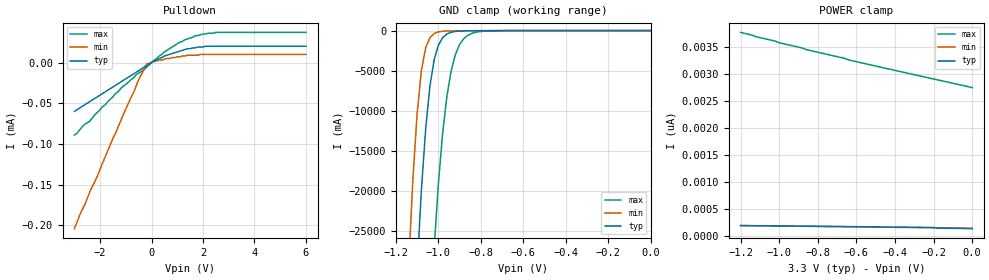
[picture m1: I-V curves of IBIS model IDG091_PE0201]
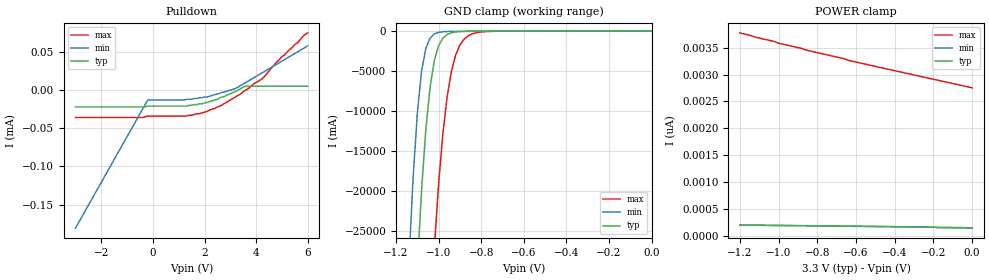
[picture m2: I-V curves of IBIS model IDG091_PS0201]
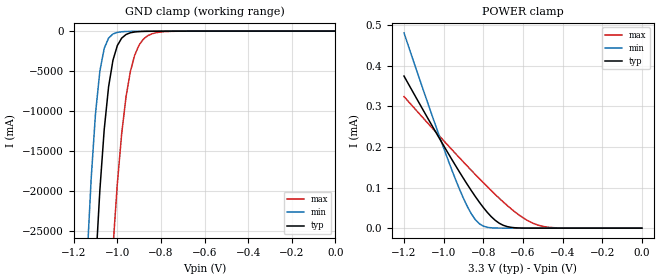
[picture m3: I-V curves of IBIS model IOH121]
| Texas Instruments Incorporated
| DAC5652A DUAL, 10-BIT 275 MSPS DIGITAL-TO-ANALOG CONVERTER
[IBIS Ver]   2.1
[File name]   dac5652a.ibs
[File Rev]   1.0
[Date]   22 FEB 2018
[Source]   Preliminary Model
[Notes]
   Technology type GS30
[Disclaimer]   Please be aware that in the absence of a written agreement
|   Texas Instruments(TI) assumes no liability for:
|   (1) The accuracy of the IBIS models provided to your company
|   (2) The proper functioning of these Models in your design
|   or for any resulting applications;or
|   property rights resulting from your use of these models.
|   TI provides IBIS Models as a service to our customers and
|   therefore reserves the right to limit distribution of the
|   Models.
[Copyright]   Property of Texas Instruments Incorporated.
|   Unauthorised reproduction and/or distribution is strictly.
|   prohibited.
|   This product is protected under copyright law and trade
|   secret law as an unpublished work.
|   (C) Copyright 2018,
|   Texas Instruments Incorporated. All Rights Reserved.
|   These commodities are under the U.S.
|   Government distribution license control.As such,they are not
|   to be re-exported without the prior approval of the U.S.
|   Department of Commerce.
|  Component DAC5652A 48-pin TQFP - PFB Package
|  Part # DAC5652A
[Component]   DAC5652A
[Manufacturer]   Texas Instruments
[Package]   |48 TQFP - PFB Package
|   typ   min   max
R_pkg   0.114   0.028   0.162
L_pkg   3.172nH   2.482nH   4.042nH
C_pkg   0.140pF   0.089pF   0.217pF
[Pin]   signal_name   model_name   R_pin   L_pin   C_pin
   1   DA9   IDG091_PE0201   0.083   3.524nH   0.213pF
   2   DA8   IDG091_PE0201   0.153   3.828nH   0.113pF
   3   DA7   IDG091_PE0201   0.147   3.682nH   0.108pF
   4   DA6   IDG091_PE0201   0.143   3.569nH   0.104pF
   5   DA5   IDG091_PE0201   0.140   3.487nH   0.103pF
   6   DA4   IDG091_PE0201   0.073   3.022nH   0.199pF
   7   DA3   IDG091_PE0201   0.139   3.401nH   0.104pF
   8   DA2   IDG091_PE0201   0.140   2.975nH   0.197pF
   9   DA1   IDG091_PE0201   0.140   3.391nH   0.098pF
   10   DA0   IDG091_PE0201   0.140   3.410nH   0.103pF
   11   NC   nc   0.141   3.461nH   0.105pF
   12   NC   nc   0.073   3.102nH   0.206pF
   13   NC   nc   0.073   3.174nH   0.211pF
   14   NC   nc   0.073   3.260nH   0.218pF
   15   DGND   GND   0.078   3.360nH   0.223pF
   16   DVDD   POWER   0.028   2.456nH   0.090pF
   17   WRTA/WRTIQ   IDG091_PE0201   0.153   3.934nH   0.103pF
   18   CLKA/CLKIQ   IDG091_PE0201   0.076   3.327nH   0.217pF
   19   CLKB/RESETIQ  IDG091_PE0201   0.076   3.233nH   0.212pF
   20   WRTB/SELECTIQ IDG091_PE0201   0.073   3.154nH   0.206pF
   21   DGND   GND   0.073   3.096nH   0.204pF
   22   DVDD   POWER   0.073   3.051nH   0.202pF
   23   DB9   IDG091_PE0201   0.073   3.018nH   0.201pF
   24   DB8   IDG091_PE0201   0.143   3.416nH   0.105pF
   25   DB7   IDG091_PE0201   0.073   2.993nH   0.198pF
   26   DB6   IDG091_PE0201   0.073   3.008nH   0.199pF
   27   DB5   IDG091_PE0201   0.141   3.462nH   0.105pF
   28   DB4   IDG091_PE0201   0.143   3.533nH   0.107pF
   29   DB3   IDG091_PE0201   0.075   3.190nH   0.210pF
   30   DB2   IDG091_PE0201   0.075   3.272nH   0.215pF
   31   DB1   IDG091_PE0201   0.153   3.839nH   0.112pF
   32   DB0   IDG091_PE0201   0.028   2.477nH   0.094pF
   33   NC   nc   0.153   2.919nH   0.089pF
   34   NC   nc   0.145   2.784nH   0.095pF
   35   NC   nc   0.140   2.700nH   0.089pF
   36   NC   nc   0.072   2.292nH   0.163pF
   37   SLEEP   IDG091_PE0201   0.072   2.270nH   0.164pF
   38   AGND   GND   0.072   2.255nH   0.163pF
   39   IOUTB1   IOH121   0.072   2.252nH   0.161pF
   40   IOUTB2   IOH121   0.140   2.675nH   0.091pF
   41   BIASJ_B   IOH121   0.140   2.662nH   0.093pF
   42   GSET   IDG091_PS0201   0.072   2.242nH   0.160pF
   43   EXTIO   IOH121   0.138   2.652nH   0.090pF
   44   BIASJ_A   IOH121   0.139   2.671nH   0.090pF
   45   IOUTA2   IOH121   0.142   2.710nH   0.091pF
   46   IOUTA1   IOH121   0.145   2.768nH   0.093pF
   47   AVDD   POWER   0.150   2.854nH   0.097pF
   48   MODE   IDG091_PS0201   0.077   2.482nH   0.163pF
| Models and submodels in the file (3): IDG091_PE0201 (Input), IDG091_PS0201 (Input), IOH121 (Input)
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[Model]   IDG091_PE0201
Model_type   Input
Polarity   Non-Inverting
| signals   A, Y
Vinl = 0.8V
Vinh = 2.0V
|   typ   min   max
C_comp   3.016p   2.9215p   3.4873p
|   typ   min   max
[Temperature Range]   25   -40.0   125
|   typ   min   max
[Voltage Range]   3.30V   3.00V   3.60V
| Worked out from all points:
|   slope of the pulldown table from 0 to 0.495 V, typ, clamps not added: 62.7 kohm
|   GND clamp passes 1 mA (typ) near -0.58 V on its own axis
[Pulldown]
|   Voltage   I(typ)   I(min)   I(max)
-3V       -60uA      -204uA     -89uA
-2.6V     -52uA      -175uA     -76uA
-2.4V     -48uA      -159uA     -72uA
-2.1V     -42uA      -139uA     -61uA
-1.1V     -22uA      -64uA      -29uA
-500mV    -10uA      -21uA      -13uA
-200mV    -4uA       -2uA       -6uA
500mV     8uA        4uA        13uA
1.1V      14uA       7uA        25uA
1.7V      18uA       9uA        33uA
2.5V      20uA       10uA       37uA
6V        20uA       10uA       37uA
[GND_clamp]
|   Voltage   I(typ)   I(min)   I(max)
-1.2V     -98.78A    -71.42A    -148.8A
-1.14V    -54.21A    -29.33A    -101.8A
-1.1V     -29.69A    -10.34A    -73.18A
-1.08V    -19.94A    -5.01A     -60A
-1.06V    -12.33A    -2.162A    -47.8A
-1.04V    -6.983A    -880.6mA   -36.79A
-1.02V    -3.664A    -361.6mA   -27.18A
-980mV    -884.2mA   -83.74mA   -12.87A
-960mV    -428mA     -53.16mA   -8.232A
-920mV    -110.2mA   -33.2mA    -3A
-880mV    -38.87mA   -25.56mA   -1.002A
0V        -427.6fA   -2.728fA   -107pA
[POWER_clamp]
|   Voltage   I(typ)   I(min)   I(max)
-1.2V     197.2pA    197.2pA    3.775nA
-1.14V    194.5pA    194.5pA    3.723nA
-1.12V    194.5pA    193.6pA    3.695nA
-1.02V    191pA      190.1pA    3.613nA
-1V       191pA      189.2pA    3.583nA
-880mV    187.4pA    184.7pA    3.485nA
-860mV    187.4pA    184.7pA    3.456nA
-660mV    178.5pA    175.9pA    3.293nA
-640mV    178.1pA    175pA      3.265nA
-200mV    160.8pA    156.8pA    2.912nA
-180mV    148.8pA    155.9pA    2.896nA
0V        139.9pA    145.7pA    2.752nA
[Model]   IDG091_PS0201
Model_type   Input
Polarity   Non-Inverting
| signals   A, Y
Vinl = 0.8V
Vinh = 2.0V
|   typ   min   max
C_comp   2.9577p   2.8282p   3.4534p
|   typ   min   max
[Temperature Range]   25   -40.0   125
|   typ   min   max
[Voltage Range]   3.30V   3.00V   3.60V
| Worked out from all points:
|   GND clamp passes 1 mA (typ) near -0.58 V on its own axis
[Pulldown]
|   Voltage   I(typ)   I(min)   I(max)
-3V       -22uA      -181uA     -36uA
-400mV    -22uA      -25uA      -36uA
-200mV    -21uA      -13uA      -34uA
1.3V      -21uA      -12uA      -34uA
1.9V      -18uA      -10uA      -30uA
2.6V      -10uA      -4uA       -21uA
3.2V      -2uA       2uA        -9uA
3.6V      5uA        10uA       0A
4.3V      5uA        24uA       17uA
5V        5uA        38uA       44uA
5.8V      5uA        54uA       70uA
6V        5uA        58uA       75uA
[GND_clamp]
|   Voltage   I(typ)   I(min)   I(max)
-1.2V     -98.78A    -71.42A    -148.8A
-1.14V    -54.21A    -29.33A    -101.8A
-1.1V     -29.69A    -10.34A    -73.18A
-1.08V    -19.94A    -5.01A     -60A
-1.06V    -12.33A    -2.162A    -47.8A
-1.04V    -6.983A    -880.6mA   -36.79A
-1.02V    -3.664A    -361.6mA   -27.18A
-980mV    -884.2mA   -83.74mA   -12.87A
-960mV    -428mA     -53.16mA   -8.232A
-920mV    -110.2mA   -33.2mA    -3A
-880mV    -38.87mA   -25.56mA   -1.002A
0V        -427.6fA   -2.728fA   -107pA
[POWER_clamp]
|   Voltage   I(typ)   I(min)   I(max)
-1.2V     197.2pA    197.2pA    3.775nA
-1.14V    194.5pA    194.5pA    3.723nA
-1.12V    194.5pA    193.6pA    3.695nA
-1.02V    191pA      190.1pA    3.613nA
-1V       191pA      189.2pA    3.583nA
-880mV    187.4pA    184.7pA    3.485nA
-860mV    187.4pA    184.7pA    3.456nA
-660mV    178.5pA    175.9pA    3.293nA
-640mV    178.1pA    175pA      3.265nA
-200mV    160.8pA    156.8pA    2.912nA
-180mV    148.8pA    155.9pA    2.896nA
0V        139.9pA    145.7pA    2.752nA
[Model]   IOH121
Model_type   Input
Polarity   Non-Inverting
| signals   Y
Vinl = 0.8V
Vinh = 2.0V
|   typ   min   max
C_comp   1.8732p   1.8084p   2.1271p
|   typ   min   max
[Temperature Range]   25   -40.0   125
|   typ   min   max
[Voltage Range]   3.30V   3.00V   3.60V
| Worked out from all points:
|   GND clamp passes 1 mA (typ) near -0.59 V on its own axis
[GND_clamp]
|   Voltage   I(typ)   I(min)   I(max)
-1.2V     -98.78A    -71.42A    -148.8A
-1.14V    -54.21A    -29.33A    -101.8A
-1.1V     -29.69A    -10.34A    -73.18A
-1.08V    -19.94A    -5.009A    -60A
-1.06V    -12.32A    -2.162A    -47.8A
-1.04V    -6.982A    -879.7mA   -36.79A
-1.02V    -3.664A    -360.7mA   -27.18A
-980mV    -883.6mA   -82.98mA   -12.87A
-960mV    -427.4mA   -52.44mA   -8.231A
-920mV    -109.8mA   -32.58mA   -3A
-880mV    -38.47mA   -25.05mA   -1.002A
0V        -6.6pA     -7.2pA     -9.285pA
[POWER_clamp]
|   Voltage   I(typ)   I(min)   I(max)
-1.2V     374.2uA    480.4uA    323.8uA
-1.04V    236.5uA    251.8uA    236.8uA
-940mV    154uA      119.8uA    183.5uA
-880mV    107.1uA    52.79uA    152.3uA
-840mV    77.73uA    20.85uA    131.9uA
-820mV    63.94uA    10.91uA    121.8uA
-760mV    28.38uA    817.7nA    92.48uA
-700mV    7.217uA    43.91nA    64.78uA
-600mV    217.9nA    452.1pA    25.71uA
-520mV    10.24nA    137.7pA    6.943uA
-420mV    349.5pA    127.9pA    575.2nA
0V        110.6pA    113.7pA    2.598nA
